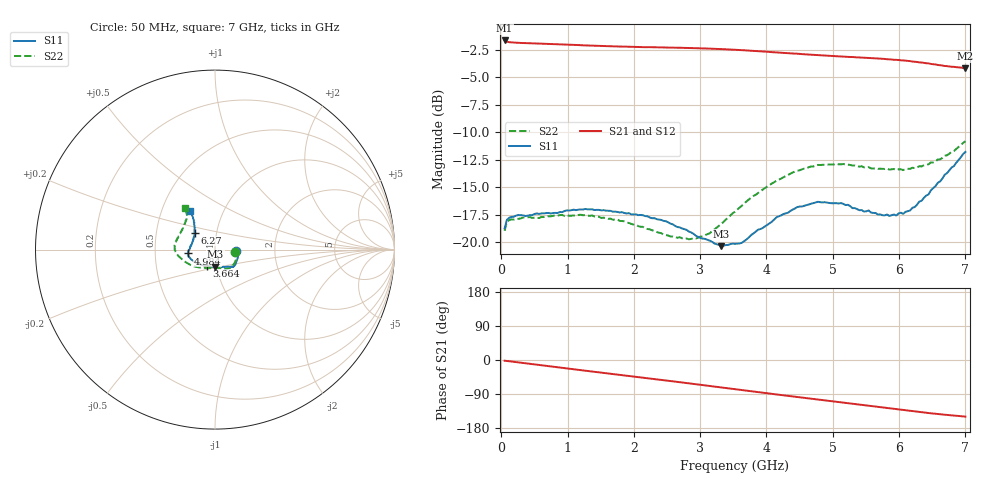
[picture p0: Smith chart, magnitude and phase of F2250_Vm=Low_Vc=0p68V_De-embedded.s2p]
! Integrated Device Technology
! Corporate Headquarters
! 6024 Silver Creek Valley Road
! San Jose, CA 95138  USA
! Phone:  1-408-284-8200
! Toll Free:  1-800-223-1366
! Webpage:  http://www.idt.com/
! Timing and RF Division
! 515 Groton Road, Suite 102
! Westford, MA 01886-6024
! Device:  F2250
! Description: Voltage Variable RF Attenuator
! Frequency:  50.0 -  6000.00 MHz
! Package:  3x3 mm Thin QFN Plastic Package: 16 pin
! Ports:  2 RF, 3 DC
!  Pin  1  = GND
!  Pin  2  = NC
!  Pin  3  = RF1  = Port 1
!  Pin  4  = NC
!  Pin  5  = GND
!  Pin  6  = GND
!  Pin  7  = GND
!  Pin  8  = GND
!  Pin  9  = NC
!  Pin 10  = RF2  = Port 2
!  Pin 11  = NC
!  Pin 12  = GND
!  Pin 13  = GND
!  Pin 14  = VCNTRL
!  Pin 15  = VDD
!  Pin 16  = VMODE
! Vcntrl:  0.680 Volts
! Vmode:  +0.000 Volts
! Vdd:  +3.30  Volts
! Current:  1.147 mA
! Data:  The device was measured on a the F2250 evaluation board which has
!  individual transmission lines to the RF pins.  Data was collected
!  using a calibrated network analyzer.  The evaluation board was
!  de-embedded using a TRL calibration technique.
!  The reference plane is the edge of the package pin.
! Misc:  SN 10
!  Action Tracker AT0258
! Date Measured:  2014-11-26
! Date:  2015-10-15  MJV
! Note:
!  Integrated Device Technology supplies this data as a sample of measured
!  data at the package pin for this product.  Your particular data for this
!  product may vary.
!  Data was taken at 25 degrees C.
!  Integrated Device Technology reserves the right to change this data at anytime.
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# GHz S dB R 50
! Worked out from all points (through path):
!   201 points, 50 MHz to 7 GHz, reference 50 ohm
!   highest |S21| = -1.67 dB at 50 MHz (marker M1); lowest = -4.2 dB at 7 GHz (marker M2)
!   group delay of S21, straight-line fit = 59.9 ps
!   lowest |S11| = -20.4 dB at 3.317 GHz (marker M3), VSWR 1.21, Z = 49.2 - j9.51 ohm
!   |S11| at or under -10 dB: start of sweep to end of sweep
!   |S22| runs from -19.8 to -10.8 dB; largest |S21 - S12| = 0.00093
!   S11 on the Smith chart (normalised r, x): 50 MHz: 1.26, -0.02; 3.664 GHz: 0.90, -0.16; 4.984 GHz: 0.74, -0.03; 6.27 GHz: 0.78, +0.15; 7 GHz: 0.70, +0.32
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0.05  -18.76 -4.4  -1.67 -1.9  -1.66 -1.9  -18.97 -6.0
0.08475  -17.97 -4.8  -1.78 -2.5  -1.78 -2.5  -18.15 -5.8
0.22375  -17.59 -8.8  -1.87 -5.5  -1.87 -5.5  -17.90 -10.8
0.71025  -17.35 -24.5  -1.98 -16.2  -1.97 -16.2  -17.65 -30.3
1.2315  -17.04 -38.2  -2.11 -27.5  -2.11 -27.5  -17.56 -49.0
1.75275  -17.26 -45.0  -2.22 -38.5  -2.21 -38.5  -17.93 -60.2
2.37825  -17.96 -49.0  -2.29 -51.7  -2.29 -51.7  -19.15 -72.3
2.7605  -18.82 -57.4  -2.34 -60.1  -2.34 -60.1  -19.72 -87.9
2.93425  -19.42 -63.8  -2.37 -63.9  -2.38 -63.9  -19.68 -98.0
3.14275  -19.86 -76.2  -2.41 -68.5  -2.41 -68.5  -19.20 -112.3
3.3165  -20.37 -89.4  -2.45 -72.4  -2.45 -72.4  -18.37 -123.0
3.525  -20.16 -106.1  -2.52 -77.1  -2.51 -77.1  -17.24 -135.0
3.664  -19.91 -117.6  -2.56 -80.2  -2.56 -80.2  -16.48 -141.5
4.1505  -17.75 -145.9  -2.76 -90.9  -2.76 -90.9  -14.43 -162.7
4.46325  -16.81 -157.7  -2.87 -97.7  -2.88 -97.7  -13.53 -172.1
4.7065  -16.46 -164.8  -2.97 -103.0  -2.97 -103.0  -13.12 -178.0
4.9845  -16.47 -171.8  -3.08 -108.9  -3.07 -108.9  -12.95 175.6
5.85325  -17.62 160.1  -3.39 -127.4  -3.39 -127.4  -13.41 155.3
6.06175  -17.43 150.6  -3.48 -131.9  -3.49 -131.9  -13.46 149.1
6.27025  -16.60 140.3  -3.62 -136.4  -3.63 -136.4  -13.21 142.4
6.61775  -14.49 127.5  -3.92 -143.1  -3.92 -143.1  -12.48 130.8
7  -11.81 122.6  -4.18 -149.3  -4.19 -149.4  -10.83 126.2
